PROGRAM MAIN
VAR
    sendToA : BOOL := FALSE; // HMI can set this

    B_DataToSend   : ST_B_To_A;
    A_DataReceived : ST_A_To_B; // PLC A writes into this variable by ADS

    SendTimer      : TON;
    OneMinutePulse : BOOL;
    SeqB           : UDINT;

    CommsSendToA   : FB_AdsSend_B_To_A;

    SendBusy       : BOOL;
    SendDone       : BOOL;
    SendError      : BOOL;
    SendErrId      : UDINT;
END_VAR

SendTimer(IN := NOT SendTimer.Q, PT := T#10S);
OneMinutePulse := SendTimer.Q;

IF OneMinutePulse AND sendToA THEN
    SeqB := SeqB + 1;

    B_DataToSend.SequenceNo  := SeqB;
    B_DataToSend.Running     := TRUE;
    B_DataToSend.ActualValue := 98.76 +  UDINT_TO_REAL(SeqB);
    B_DataToSend.AlarmCode   := UDINT_TO_INT(SeqB);	
	B_DataToSend.Hello := CONCAT(
    'Hello from B to A  with Sequence ',
    UDINT_TO_STRING(B_DataToSend.SequenceNo)
);	
END_IF

CommsSendToA(
    xExecute       := OneMinutePulse AND sendToA,
    sRemoteNetId   := '10.10.1.2.1.1',
    nRemoteAdsPort := 851,
    sRemoteSymbol  := 'MAIN.B_DataReceived',
    stData         := B_DataToSend,
    xBusy          => SendBusy,
    xDone          => SendDone,
    xError         => SendError,
    nErrId         => SendErrId
);

END_PROGRAM
